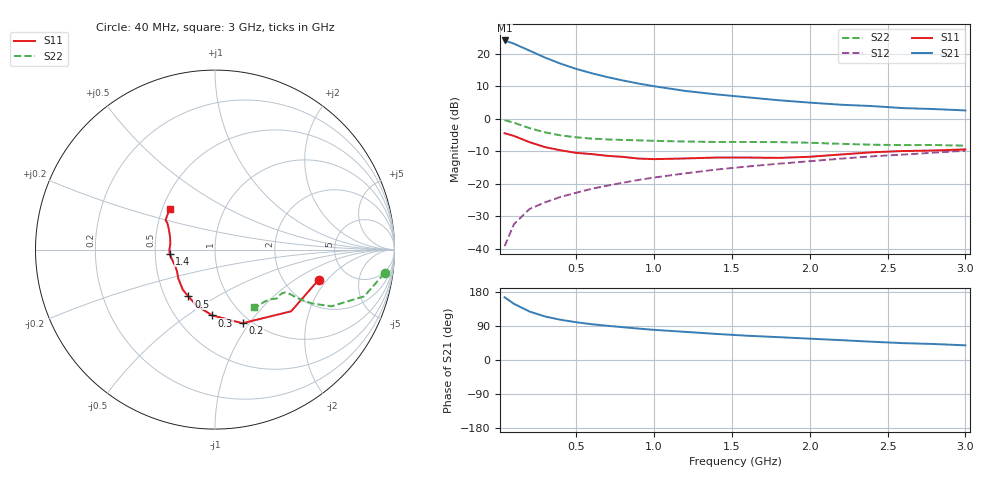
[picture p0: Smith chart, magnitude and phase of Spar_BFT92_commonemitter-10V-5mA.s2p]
! Filename:  BFT92G.S2P  Version:  2.0
! NXP part #: BFT92  Date: May 1990
! Bias condition: Vce=-10V, Ic=-5mA
#  MHz  S  MA  R  50
! Freq  S11  S21  S12  S22  !GUM [dB]
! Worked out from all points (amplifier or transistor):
!   21 points, 40 MHz to 3 GHz, reference 50 ohm
!   highest |S21| = 24.1 dB at 40 MHz (marker M1)
!   |S21| within 3 dB of that: start of sweep to 194.2 MHz
!   unconditionally stable (mu >= 1): 836.8 MHz to 2.557 GHz
!   at 300 MHz: K = 0.70, MSG = 22.3 dB, |S12| = -25.7 dB
!   at 1 GHz: K = 1.04, MAG = 12.9 dB, |S12| = -18.1 dB
!   at 3 GHz: K = 0.96, MSG = 6.2 dB, |S12| = -9.8 dB
!   S11 on the Smith chart (normalised r, x): 40 MHz: 3.08, -1.63; 200 MHz: 0.91, -0.93; 300 MHz: 0.74, -0.63; 500 MHz: 0.66, -0.38; 1.4 GHz: 0.60, -0.03; 3 GHz: 0.55, +0.28
40  0.601 -16.3  16.07 165.5  0.011 82.4  0.954 -7.9
100  0.546 -39.0  14.32 148.3  0.024 73.8  0.871 -17.4
200  0.438 -69.5  11.22 127.9  0.041 66.4  0.721 -26.0
300  0.367 -92.4  8.755 114.8  0.052 64.7  0.619 -29.0
400  0.328 -108.3  7.064 106.1  0.063 65.0  0.557 -30.2
500  0.3 -119.6  5.868 99.7  0.073 65.5  0.52 -30.5
600  0.287 -128.5  5.029 94.4  0.084 66.3  0.497 -30.6
700  0.27 -135.8  4.389 90.3  0.094 67.3  0.482 -30.7
800  0.26 -141.9  3.896 86.5  0.104 67.8  0.474 -30.9
900  0.245 -149.5  3.493 82.9  0.115 68.1  0.467 -31.1
1000  0.24 -156.2  3.176 79.5  0.125 68.2  0.459 -31.4
1200  0.246 -167.5  2.691 74.3  0.145 68.3  0.448 -32.7
1400  0.254 -175.0  2.38 68.8  0.166 68.2  0.441 -34.8
1600  0.254 179.8  2.144 64.0  0.185 67.7  0.441 -36.7
1800  0.251 172.3  1.934 60.3  0.204 67.7  0.439 -38.3
2000  0.261 163.8  1.777 56.3  0.223 67.1  0.429 -39.8
2200  0.283 155.7  1.65 52.4  0.244 66.5  0.413 -42.1
2400  0.306 150.5  1.573 48.2  0.265 65.6  0.4 -46.7
2600  0.32 149.4  1.464 44.5  0.282 64.8  0.395 -50.8
2800  0.326 145.2  1.414 42.2  0.302 64.6  0.396 -53.3
3000  0.339 138.1  1.348 38.7  0.324 63.7  0.387 -55.6
